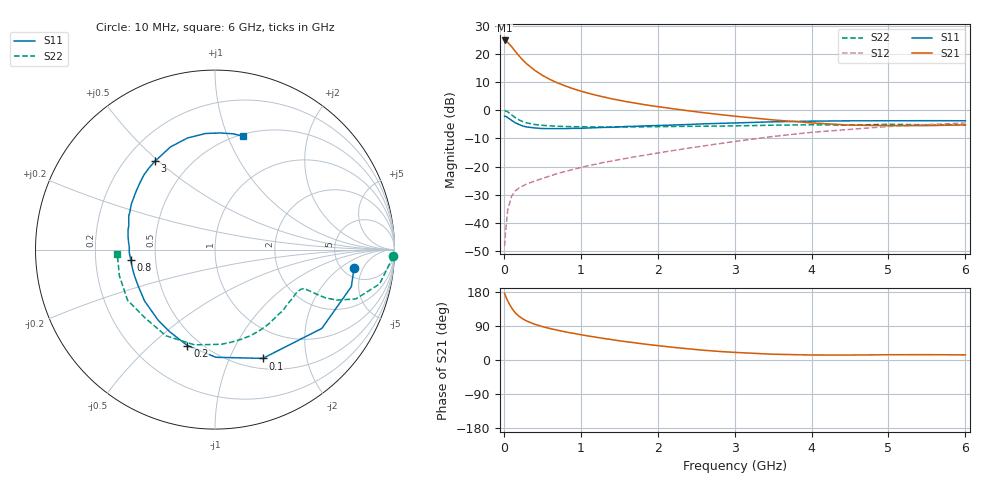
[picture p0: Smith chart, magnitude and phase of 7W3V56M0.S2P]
! Infineon Technologies  Discrete & RF Semiconductors
! BFS17W
! Si NPN RF Bipolar Junction Transistor in SOT323
! VCE = 3.5 V  IC = 6 mA
! Common Emitter S-Parameters:  August  1999
# GHz  S  MA  R  50
!  f  S11  S21  S12  S22
! GHz  MAG  ANG  MAG  ANG  MAG  ANG  MAG  ANG
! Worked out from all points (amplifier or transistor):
!   36 points, 10 MHz to 6 GHz, reference 50 ohm
!   highest |S21| = 24.7 dB at 10 MHz (marker M1)
!   |S21| within 3 dB of that: start of sweep to 123.8 MHz
!   unconditionally stable (mu >= 1): 502.3 MHz to 2.675 GHz; 4.371 GHz to end of sweep
!   at 250 MHz: K = 0.64, MSG = 22.2 dB, |S12| = -26.8 dB
!   at 1.4 GHz: K = 1.24, MAG = 8.1 dB, |S12| = -18.0 dB
!   at 6 GHz: K = 1.07, MAG = -2.0 dB, |S12| = -4.5 dB
!   S11 on the Smith chart (normalised r, x): 10 MHz: 6.37, -3.33; 100 MHz: 0.62, -1.34; 200 MHz: 0.43, -0.66; 800 MHz: 0.36, -0.05; 3 GHz: 0.32, +0.49; 6 GHz: 0.52, +1.14
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0.01  0.7813 -7.5  17.24 175.5  0.0039 84.1  0.9932 -2.1
0.02  0.7873 -15.2  17.16 170.0  0.0064 88.6  0.9734 -5.0
0.05  0.7397 -36.4  16.05 155.9  0.017 72.0  0.9367 -11.8
0.1  0.662 -66.3  13.41 137.6  0.0299 61.0  0.8314 -19.3
0.15  0.5999 -89.6  11 124.1  0.0373 54.0  0.7351 -22.5
0.2  0.5565 -106.0  9.1 115.0  0.0423 51.2  0.6705 -23.6
0.25  0.5229 -118.8  7.66 108.1  0.0458 49.4  0.6251 -23.7
0.3  0.5051 -128.8  6.586 102.7  0.0496 49.4  0.5957 -23.6
0.4  0.4857 -143.9  5.117 94.4  0.0554 51.0  0.5586 -23.6
0.5  0.4738 -154.1  4.171 88.2  0.062 53.0  0.54 -23.8
0.6  0.4719 -161.7  3.508 83.0  0.0685 55.5  0.5284 -24.6
0.8  0.4725 -173.2  2.69 74.2  0.0823 58.4  0.515 -27.6
0.9  0.4778 -177.8  2.405 70.5  0.0893 59.8  0.5112 -29.2
1.1  0.4854 174.0  1.999 63.2  0.1044 61.4  0.5083 -33.4
1.3  0.4967 167.1  1.716 56.8  0.119 63.1  0.5054 -38.1
1.6  0.5158 158.6  1.416 48.0  0.1411 64.5  0.5052 -45.6
2.2  0.547 143.3  1.062 33.5  0.1931 66.5  0.5156 -62.3
3  0.595 124.3  0.785 20.1  0.2795 64.6  0.5287 -86.2
3.5  0.6234 113.5  0.674 15.2  0.343 60.9  0.5429 -102.2
4.5  0.649 94.6  0.544 13.1  0.458 48.8  0.5447 -135.5
5.5  0.6531 81.0  0.534 14.1  0.5564 36.2  0.5523 -164.7
6  0.6511 76.0  0.55 13.5  0.5949 30.0  0.5449 -177.6
